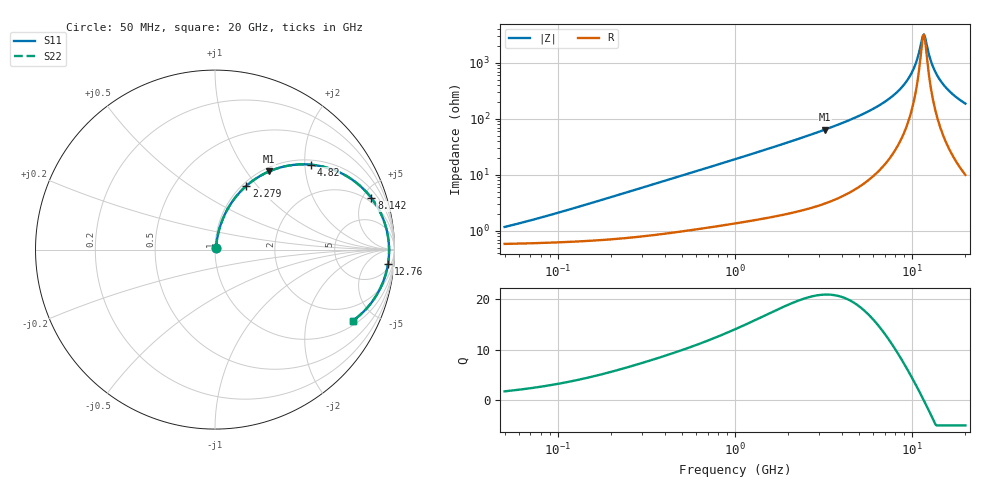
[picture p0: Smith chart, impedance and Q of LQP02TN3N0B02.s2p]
!Murata Part Number: LQP02TN3N0B02
!These Parameters are Measured in Series Mode Connection
!  o--[Z]--o
!Port1  Port2
!  o-------o
!Freq. Start=50[MHz] Stop=20[GHz], 401[Steps]
# Hz S RI R 50
!Freq.(Hz) S11(Real) S11(Imag) S21(Real) S21(Imag) S12(Real) S12(Imag) S22(Real) S22(Imag)
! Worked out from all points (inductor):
!   401 points, 50 MHz to 20 GHz, reference 50 ohm
!   read as one part in series: L = 3.19 nH near 92.4 MHz
!   highest Q = 20.9 at 3.217 GHz (marker M1), where L = 3.18 nH
!   self-resonance near 11.49 GHz
!   S11 on the Smith chart (normalised r, x): 50 MHz: 1.01, +0.02; 2.279 GHz: 1.04, +0.88; 4.82 GHz: 1.11, +2.14; 8.142 GHz: 1.60, +5.81; 12.76 GHz: 8, -21; 20 GHz: 1.20, -3.75
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5e7  0.00592 0.0101  0.9941 -0.0101  0.9941 -0.0101  0.00592 0.0101
1.364002e8  0.00722 0.0269  0.9928 -0.0269  0.9928 -0.0269  0.00722 0.0269
3.721004e8  0.0137 0.0709  0.9863 -0.0709  0.9863 -0.0709  0.0137 0.0709
1e9  0.0469 0.1788  0.9531 -0.1788  0.9531 -0.1788  0.0469 0.1788
2.279204e9  0.1743 0.3548  0.8257 -0.3548  0.8257 -0.3548  0.1743 0.3548
2.728004e9  0.2329 0.399  0.7671 -0.399  0.7671 -0.399  0.2329 0.399
3.216634e9  0.3014 0.4355  0.6986 -0.4355  0.6986 -0.4355  0.3014 0.4355
4.81993e9  0.5326 0.4733  0.4674 -0.4733  0.4674 -0.4733  0.5326 0.4733
6.125241e9  0.6967 0.4289  0.3033 -0.4289  0.3033 -0.4289  0.6967 0.4289
7.442007e9  0.8224 0.3422  0.1776 -0.3422  0.1776 -0.3422  0.8224 0.3422
8.141811e9  0.8718 0.2869  0.1282 -0.2869  0.1282 -0.2869  0.8718 0.2869
9.178299e9  0.9245 0.2  0.0755 -0.2  0.0755 -0.2  0.9245 0.2
1.004137e10  0.9517 0.1272  0.0483 -0.1272  0.0483 -0.1272  0.9517 0.1272
1.066139e10  0.9633 0.0762  0.0367 -0.0762  0.0367 -0.0762  0.9633 0.0762
1.131968e10  0.9692 0.024  0.0308 -0.024  0.0308 -0.024  0.9692 0.024
1.149051e10  0.9698 0.0108  0.0302 -0.0108  0.0302 -0.0108  0.9698 0.0108
1.183995e10  0.9699 -0.0155  0.0301 0.0155  0.0301 0.0155  0.9699 -0.0155
1.276073e10  0.9638 -0.0811  0.0362 0.0811  0.0362 0.0811  0.9638 -0.0811
1.375312e10  0.9489 -0.145  0.0511 0.145  0.0511 0.145  0.9489 -0.145
1.504638e10  0.9201 -0.2175  0.0799 0.2175  0.0799 0.2175  0.9201 -0.2175
1.721783e10  0.8573 -0.3135  0.1427 0.3135  0.1427 0.3135  0.8573 -0.3135
2e10  0.7671 -0.3969  0.2329 0.3969  0.2329 0.3969  0.7671 -0.3969
